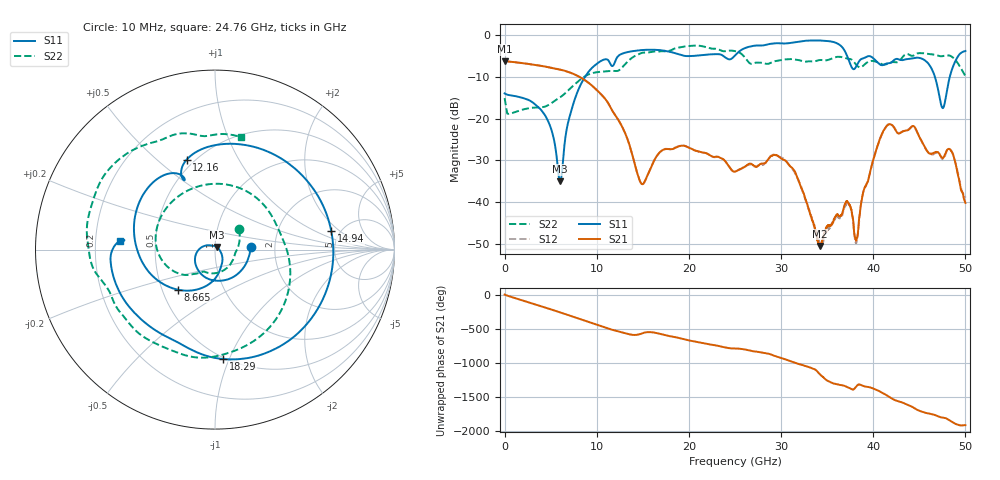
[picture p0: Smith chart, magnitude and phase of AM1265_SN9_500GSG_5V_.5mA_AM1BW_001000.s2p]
!Keysight Technologies,N5245B,MY58422270,A.16.20.02
!Date: Thursday, March 05, 2026 00:31:52
!Correction: S11(C  2-Port  )
!S21(C  2-Port  )
!S12(C  2-Port  )
!S22(C  2-Port  )
!S2P File: Measurements: S11, S21, S12, S22:
# Hz S  dB  R 50
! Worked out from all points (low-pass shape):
!   3201 points, 10 MHz to 50 GHz, reference 50 ohm
!   highest |S21| = -6.32 dB at 10 MHz (marker M1); lowest = -50.4 dB at 34.19 GHz (marker M2)
!   |S21| within 3 dB of the highest: start of sweep to 7.44 GHz
!   lowest |S11| = -34.9 dB at 6.04 GHz (marker M3), VSWR 1.04, Z = 50.9 + j1.54 ohm
!   |S11| at or under -10 dB: start of sweep to 8.75 GHz; 46.68 GHz to 48.31 GHz (1.628 GHz wide, 3.43 % of centre)
!   |S22| runs from -18.9 to -2.6 dB; largest |S21 - S12| = 0.005
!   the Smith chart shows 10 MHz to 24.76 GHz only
!   S11 on the Smith chart (normalised r, x): 10 MHz: 1.50, +0.04; 8.665 GHz: 0.60, -0.29; 12.16 GHz: 0.45, +0.63; 14.94 GHz: 4.24, +1.51; 18.29 GHz: 0.49, -0.95; 24.76 GHz: 0.31, +0.04
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1e7  -14.01 4.1  -6.32 3.5  -6.39 3.1  -15.14 40.2
2.306416e9  -15.30 -93.0  -6.89 -98.2  -6.89 -98.2  -17.69 -85.8
4.149797e9  -18.43 -157.9  -7.51 -176.5  -7.51 -176.5  -17.28 -116.4
6.040044e9  -34.94 57.7  -8.33 100.8  -8.33 100.9  -14.92 -130.9
8.352081e9  -11.52 -120.7  -10.35 -5.7  -10.34 -5.7  -10.49 -167.6
8.664519e9  -10.30 -133.2  -10.78 -20.2  -10.77 -20.2  -10.01 -176.0
1.216382e10  -5.59 107.6  -19.67 -171.9  -19.66 -171.9  -8.69 26.1
1.494451e10  -3.66 8.9  -35.66 153.3  -35.75 152.2  -4.32 -98.4
1.667854e10  -3.65 -43.5  -28.46 151.0  -28.44 151.1  -4.01 -142.2
1.828759e10  -4.27 -85.7  -27.26 102.2  -27.17 102.7  -3.48 -167.6
2.158381e10  -4.85 -143.9  -28.15 8.1  -28.18 8.6  -2.81 131.3
2.475505e10  -5.51 174.8  -32.48 -68.7  -32.59 -69.0  -3.83 77.1
2.5005e10  -4.96 173.3  -32.66 -69.0  -32.70 -68.9  -3.92 71.2
2.948848e10  -2.04 96.0  -28.76 172.1  -28.76 173.6  -6.27 -18.7
3.334708e10  -1.38 35.5  -44.07 -1.3  -43.95 -1.5  -6.38 -127.7
3.419066e10  -1.38 21.0  -50.40 -84.2  -49.11 -72.4  -6.04 -145.3
3.712758e10  -4.84 -40.5  -39.76 84.9  -40.24 88.5  -5.68 157.3
3.818986e10  -7.44 -22.4  -48.90 93.8  -49.37 91.8  -7.27 139.3
4.167354e10  -6.83 -54.5  -21.42 -57.1  -21.29 -57.6  -6.83 114.1
4.507911e10  -5.58 -102.0  -24.73 89.2  -24.70 88.3  -4.38 75.3
4.770358e10  -16.84 70.5  -28.99 -10.0  -29.29 -10.0  -5.04 40.6
5e10  -3.89 -73.4  -40.13 -118.7  -38.87 -136.5  -9.86 5.1
